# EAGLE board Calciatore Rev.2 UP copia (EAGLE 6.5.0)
Robot Calciatore SMD V2 Costruttori: Fabio Ricci Alessio Di Brigida
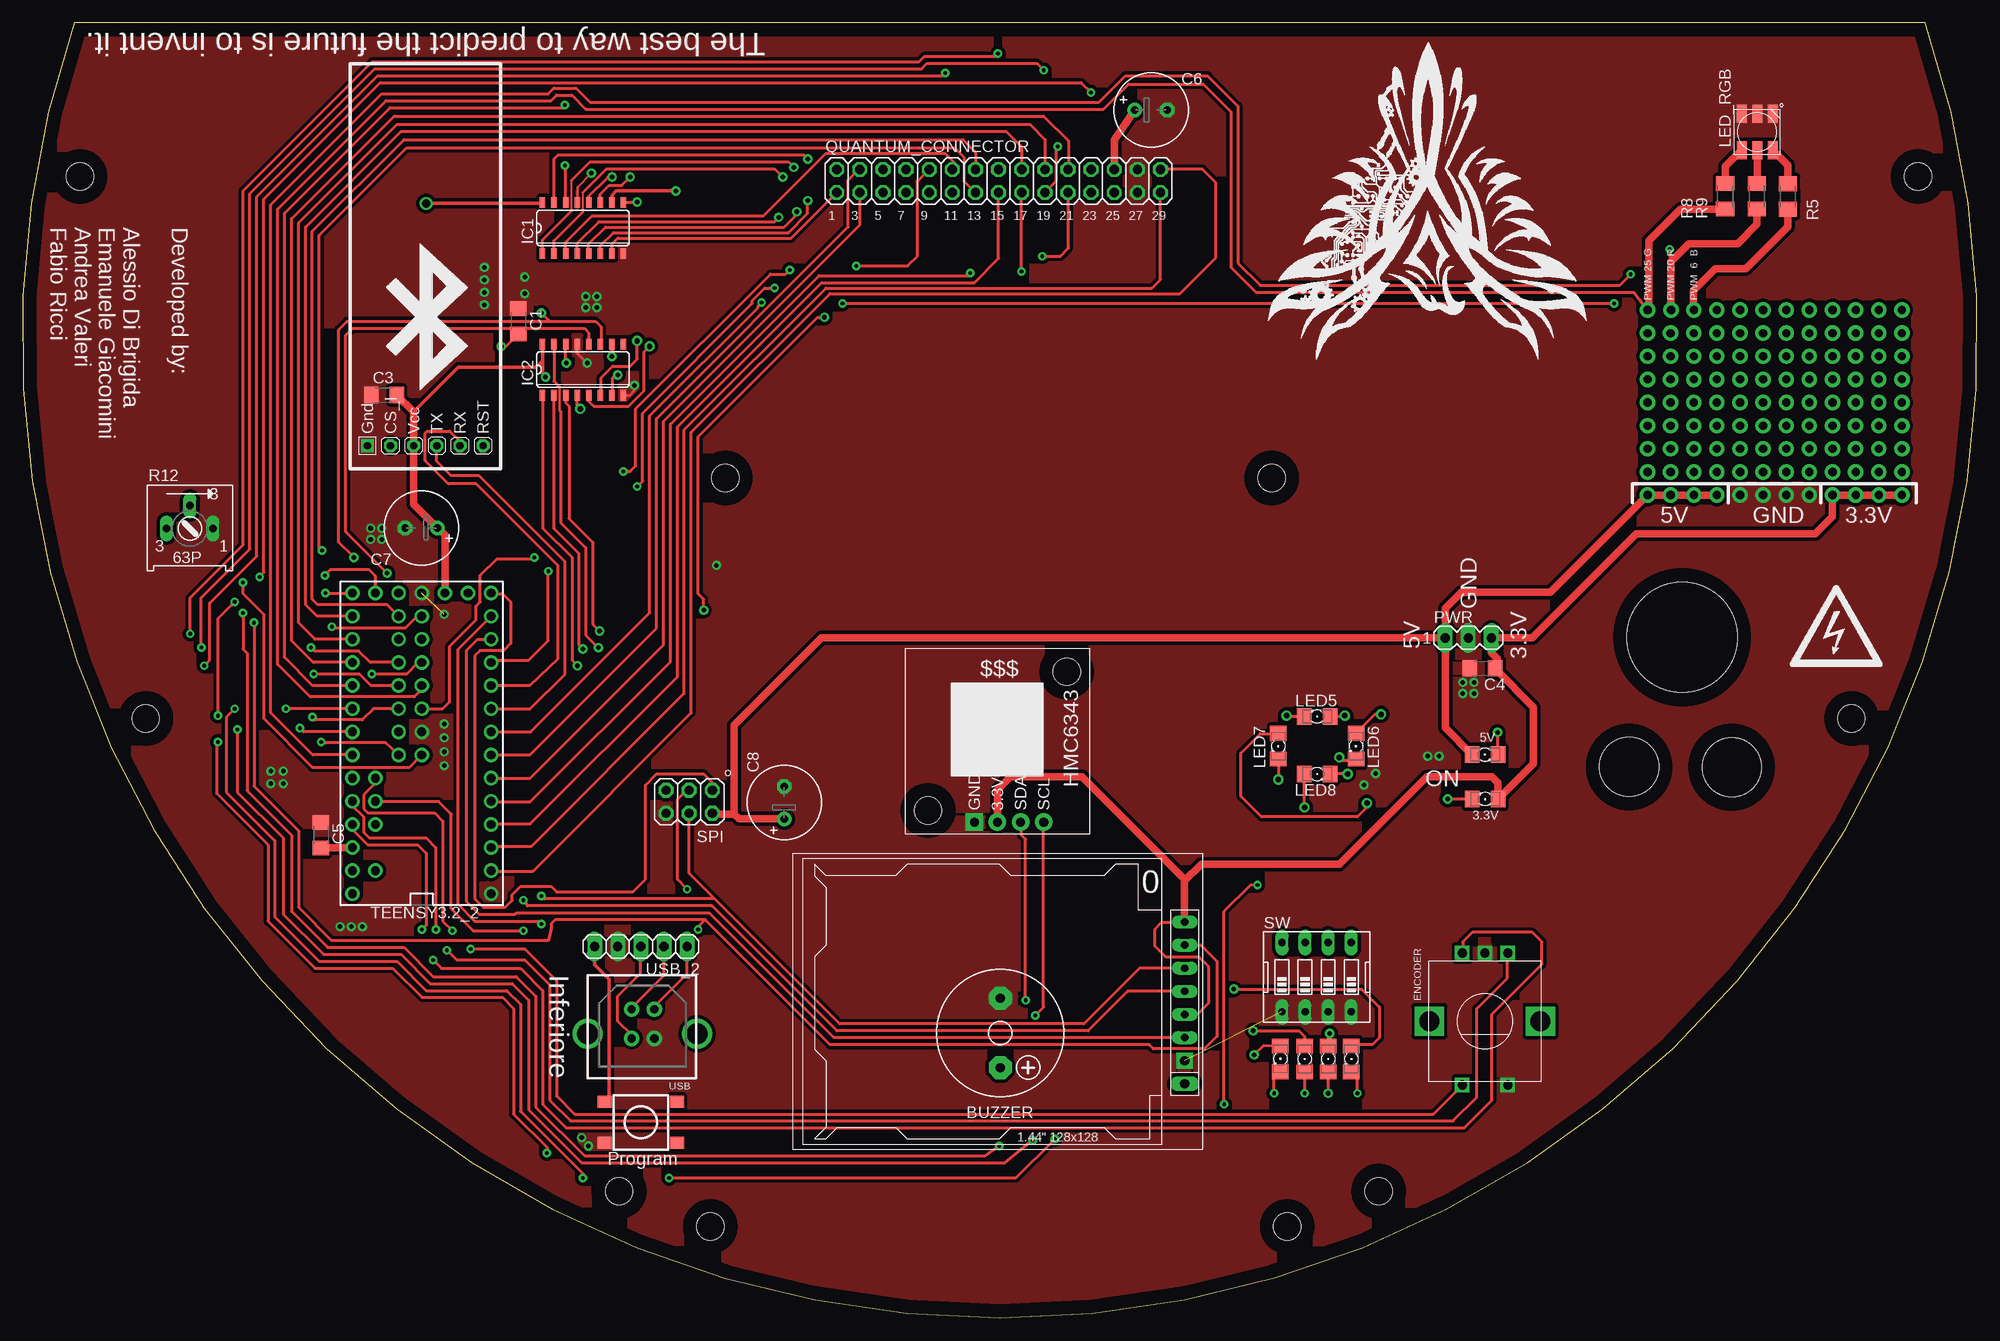
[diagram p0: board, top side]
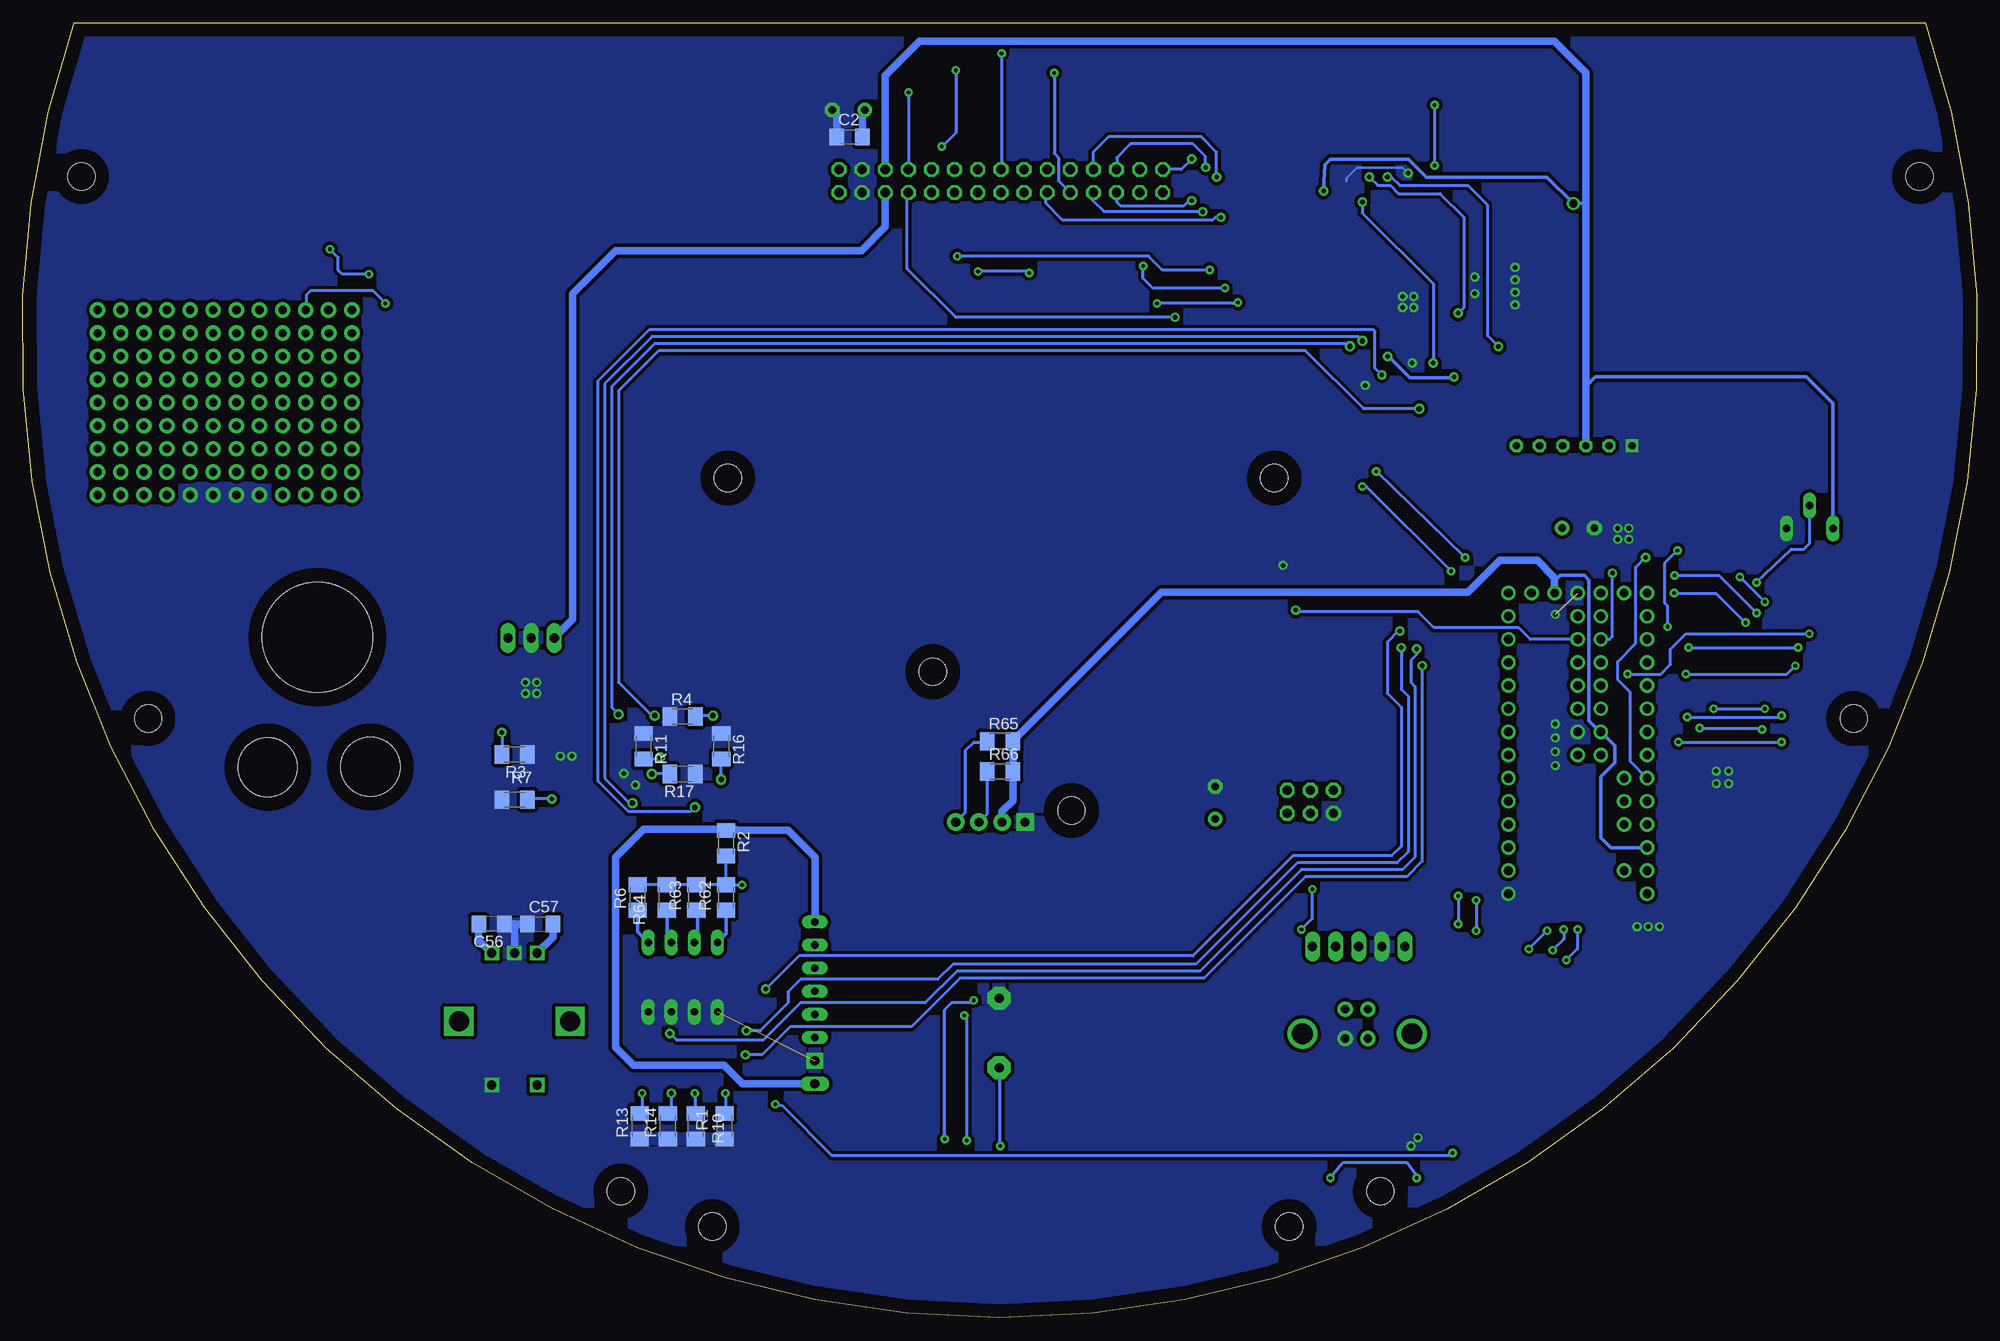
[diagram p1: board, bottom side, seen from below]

Size 214.58 x 142.18 mm. Coordinates in mm from the lower left corner, seen from the top.
Outline: 107.29,0.02 arc109 208.94,142.18 5.64,142.18 arc109 107.29,0
Copper layers (1*16): Top 0.035mm / dielectric 1.5mm / Bottom 0.035mm
Design rules "SparkFun *": minimum track width 6mil, minimum drill 8mil, track to track 6mil, track to pad 6mil, pad to pad 6mil, via to via 6mil, smd to smd 6mil, copper to edge 1.5mm, drill to drill 6mil, minimum pad ring 12mil, minimum via ring 10mil, stop-mask expansion 4mil, vias tented up to drill 25mil, thermal gap 0mil
Net classes: 0 default: width 0.254 mm, drill 0.254 mm, clearance 0.203 mm; 1 power: width 1.016 mm, drill 0.889 mm, clearance 0.508 mm; 2 gnd: width 0.864 mm, drill 0.406 mm, clearance 0.381 mm; 3 power usb: width 0.305 mm, drill 0.406 mm, clearance 0.203 mm
Holes 3 mm at 13.52,65.8 6.28,125.31 77.14,92.19 137.16,92.19 208.13,125.31 200.82,65.8 148.9,13.88 138.86,10.02 75.52,10.02 65.48,13.88
Holes 6.5 mm at 176.41,60.49 187.68,60.44
Holes 12.1 mm at 182.22,74.72

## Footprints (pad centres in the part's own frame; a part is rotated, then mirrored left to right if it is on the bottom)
F/CM12P = drill 1.016 pad 2.54 octagon: + 3.81,0; - -3.81,0
C1206 = smd 1.6 x 1.8: 1 -1.4,0; 2 1.4,0
E3,5-8 = drill 0.813 pad 1.6: + -1.778,0 | drill 0.813 pad 1.6 octagon: - 1.778,0
DISPLAY128X128 = drill 0.8 long: CS 20.32,-5.08; DC 20.32,0; LED 20.32,7.62; RST 20.32,-2.54; SCK 20.32,5.08; SDA 20.32,2.54 | drill 1 pad 1.778 square: GND 20.32,-7.62 | drill 1 long: VCC 20.32,-10.16
ALPS_EC12E_SW = drill 1 square: A -2.5,-7.5; B 2.5,-7.5; C 0,-7.5; D -2.5,7; E 2.5,7 | drill 2.2 square: GND1 -6.1,0; GND2 6.1,0
SO16 = smd 0.6 x 1.2: 1 -4.445,-2.8; 2 -3.175,-2.8; 3 -1.905,-2.8; 4 -0.635,-2.8; 5 0.635,-2.8; 6 1.905,-2.8; 7 3.175,-2.8; 8 4.445,-2.8; 9 4.445,2.8; 10 3.175,2.8; 11 1.905,2.8; 12 0.635,2.8; 13 -0.635,2.8; 14 -1.905,2.8; 15 -3.175,2.8; 16 -4.445,2.8
1206 = smd 1.6 x 1.803: A -1.422,0; C 1.422,0
RGBLED5050 = smd 2 x 1.1: 1 -2,1.7; 2 -2,0; 3 -2,-1.7; 4 2,-1.7; 5 2,0; 6 2,1.7
TACTILE_SWITCH_TALL = smd 1.55 x 1.3: A1 -3.975,-2.25; A2 3.975,-2.25; B1 -3.975,2.25; B2 3.975,2.25
MA03-1 = drill 1.016 long: 1 -2.54,0; 2 0,0; 3 2.54,0
2X15 = drill 1.016 octagon: 1 -17.78,-1.27; 2 -17.78,1.27; 3 -15.24,-1.27; 4 -15.24,1.27; 5 -12.7,-1.27; 6 -12.7,1.27; 7 -10.16,-1.27; 8 -10.16,1.27; 9 -7.62,-1.27; 10 -7.62,1.27; 11 -5.08,-1.27; 12 -5.08,1.27; 13 -2.54,-1.27; 14 -2.54,1.27; 15 0,-1.27; 16 0,1.27; 17 2.54,-1.27; 18 2.54,1.27; 19 5.08,-1.27; 20 5.08,1.27; 21 7.62,-1.27; 22 7.62,1.27; 23 10.16,-1.27; 24 10.16,1.27; 25 12.7,-1.27; 26 12.7,1.27; 27 15.24,-1.27; 28 15.24,1.27; 29 17.78,-1.27; 30 17.78,1.27
M1206 = smd 1.6 x 2: 1 -1.4,0; 2 1.4,0
S63P = drill 0.813 long: A 2.54,0; E -2.54,0; S 0,2.54
2X03 = drill 1.016 octagon: 1 -2.54,-1.27; 2 -2.54,1.27; 3 0,-1.27; 4 0,1.27; 5 2.54,-1.27; 6 2.54,1.27
EDG-04 = drill 0.813 long: 1 -3.81,-3.81; 2 -1.27,-3.81; 3 1.27,-3.81; 4 3.81,-3.81; 5 3.81,3.81; 6 1.27,3.81; 7 -1.27,3.81; 8 -3.81,3.81
TEENSY3_ALL_PINS_&_PADS = drill 0.965: 0 -7.62,13.97; 1 -7.62,11.43; 2 -7.62,8.89; 3 -7.62,6.35; 3.3V 7.62,11.43; 3.3V1 -2.54,-16.51; 3.3V2 2.54,-1.27; 4 -7.62,3.81; 5 -7.62,1.27; 6 -7.62,-1.27; 7 -7.62,-3.81; 8 -7.62,-6.35; 9 -7.62,-8.89; 10 -7.62,-11.43; 11 -7.62,-13.97; 12 -7.62,-16.51; 13 7.62,-16.51; 14/A0 7.62,-13.97; 15/A1 7.62,-11.43; 16/A2 7.62,-8.89; 17/A3 7.62,-6.35; 18/A4 7.62,-3.81; 19/A5 7.62,-1.27; 20/A6 7.62,1.27; 21/A7 7.62,3.81; 22/A8 7.62,6.35; 23/A9 7.62,8.89; 24 0,-3.81; 25 0,-6.35; 26 0,-8.89; 27 0,-11.43; 28 0,-13.97; 29 2.54,-13.97; 30 2.54,-11.43; 31 2.54,-8.89; 32 2.54,-6.35; 33 2.54,-3.81; A10 5.08,6.35; A11 5.08,3.81; A12 0,1.27; A13 2.54,1.27; AGND 7.62,13.97; AREF 5.08,8.89; GND -7.62,16.51; GND1 0,-16.51; GND2 0,-1.27; PGM 2.54,-16.51; RESET/DAC 5.08,-16.51; VBAT -5.08,-16.51; VIN 7.62,16.51; VUSB 5.08,13.97
HMC6343 = drill 1 pad 1.93: 3.3 10.16,1.27; SCL 15.24,1.27; SDA 12.7,1.27 | drill 1 pad 1.93 square: GND 7.62,1.27 | hole 3: 2.54,2.54; 17.78,17.78
BLUETOOTH = drill 0.8 pad 1.422 octagon: CS_I -3.81,-5.08; RST 6.35,-5.08; RX 3.81,-5.08; TX 1.27,-5.08; VCC -1.27,-5.08 | drill 0.8 pad 1.422 square: GND -6.35,-5.08
USB-B-PTH-VERTICAL = drill 0.914 pad 1.676: D+ 4.826,4.394; D- 4.826,7.595; GND 7.315,4.394; VBUS 7.315,7.595 | drill 2.286: P$1 0,4.902; P$2 12.04,4.902
1X05 = drill 1.016 long: 1 -5.08,0; 2 -2.54,0; 3 0,0; 4 2.54,0; 5 5.08,0

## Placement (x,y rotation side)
BUZZER  F/CM12P  [F/CM12P]  107.36,31.27 270 top
C1  [C1206]  54.44,109.41 270 top
C2  [C1206]  123.78,129.66 0 bottom
C3  [C1206]  39.68,101.31 0 top
C4  [C1206]  160.3,71.31 0 top
C5  [C1206]  32.74,53 270 top
C6  [E3,5-8]  123.9,132.6 0 top
C7  [E3,5-8]  43.77,86.71 180 top
C8  [E3,5-8]  83.62,56.56 90 top
C56  [C1206]  163.1,43.22 180 bottom
C57  [C1206]  157.76,43.22 0 bottom
DISPLAY1  DISPLAY128X128  [DISPLAY128X128]  107.28,35.84 0 top
ENCODER  EC12E_SW  [ALPS_EC12E_SW]  160.58,32.55 180 top
HIGHVOLTAGE  LOGO  [LOGOHV]  198.68,75 0 top
IC1  74LS595D  [SO16]  61.52,119.65 0 top
IC2  74LS595D  [SO16]  61.52,104.11 0 top
LED1  [1206]  140.77,28.41 270 top
LED2  [1206]  138.11,28.43 270 top
LED3  [1206]  143.36,28.41 270 top
LED4  [1206]  145.9,28.41 270 top
LED5  [1206]  142.14,66.01 180 top
LED6  [1206]  146.41,62.75 270 top
LED7  [1206]  137.87,62.75 270 top
LED8  [1206]  142.14,59.71 0 top
LED_3.3  [1206]  160.59,56.94 180 top
LED_5  [1206]  160.58,61.84 0 top
LED_RGB  [RGBLED5050]  190.47,130.19 90 top
PROGRAM  SWITCH-MOMENTARY-2SMD-4  [TACTILE_SWITCH_TALL]  67.87,21.45 180 top
PWR  [MA03-1]  158.75,74.64 0 top
QUANTUM_CONNECTOR  [2X15]  107.17,124.81 0 top
R1  1K  [M1206]  137.51,21.02 90 bottom
R2  10K  [M1206]  137.34,52.11 270 bottom
R3  1K  [M1206]  160.58,61.84 180 bottom
R4  1K  [M1206]  142.14,66.01 0 bottom
R5  1K  [M1206]  193.83,123.11 270 top
R6  10K  [M1206]  147.07,46.14 90 bottom
R7  1K  [M1206]  160.56,56.89 0 bottom
R8  1K  [M1206]  186.95,123.11 270 top
R9  1K  [M1206]  190.44,123.13 270 top
R10  1K  [M1206]  140.67,21.02 90 bottom
R11  1K  [M1206]  146.41,62.75 270 bottom
R12  [S63P]  18.34,86.66 0 top
R13  1K  [M1206]  146.84,21.02 90 bottom
R14  1K  [M1206]  143.74,21.02 90 bottom
R16  1K  [M1206]  137.87,62.75 270 bottom
R17  1K  [M1206]  142.14,59.71 180 bottom
R62  10K  [M1206]  137.34,46.14 90 bottom
R63  10K  [M1206]  140.62,46.14 270 bottom
R64  10K  [M1206]  143.84,46.14 270 bottom
R65  3.3K  [M1206]  107.27,63.31 0 bottom
R66  3.3K  [M1206]  107.24,59.99 0 bottom
SPI  [2X03]  73.18,56.66 180 top
SW  [EDG-04]  142.09,37.41 0 top
TEENSY3.2_2  TEENSY_3.1_ALL_PINS_AND_PADS  [TEENSY3_ALL_PINS_&_PADS]  43.82,63.06 180 top
U$1  [PHOENIX]  153.96,119.77 180 top
U$5  HMC6343  [HMC6343]  96.88,53.15 0 top
U$9  BLUETOOTH  [BLUETOOTH]  44.2,100.83 0 top
USB  USBPTH-VERTICAL  [USB-B-PTH-VERTICAL]  62.03,26.28 0 top
USB_2  [1X05]  67.87,40.76 180 top

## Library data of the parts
BUZZER = buzzer; OC_FARNELL: unknown; OC_NEWARK: unknown
C1-C5 C56 C57 R2 R6 R62-R66 = rcl
C6-C8 LED1-LED8 LED_3.3 LED_5 LED_RGB = adafruit
DISPLAY1 = Display 128x128
ENCODER = switch-alps; MPN: EC12E2424407; OC_FARNELL: 1520813; OC_NEWARK: 74M1068
HIGHVOLTAGE = Loghi
IC1 IC2 = SparkFun-DigitalIC; PROD_ID: IC-07875
PROGRAM = SparkFun-Electromechanical; PROD_ID: SWCH-11966
PWR = con-lstb; OC_FARNELL: unknown; OC_NEWARK: unknown
QUANTUM_CONNECTOR SPI USB_2 = pinhead
R1 R3-R5 R7-R11 R13 R14 R16 R17 = resistor
R12 = pot
SW = special
TEENSY3.2_2 = Teensy_3_and_LC_Series_Boards_v1.1
U$1 = Phoenix
U$5 = HMC6343
U$9 = Bluetooth
USB = SparkFun-Connectors

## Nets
3.3V [power]: C2.2 C3.2 C4.2 C5.2 C6.+ C7.+ DISPLAY1.LED DISPLAY1.RST DISPLAY1.VCC IC1.10 IC1.16 IC2.10 IC2.16 LED_3.3.A PWR.3 QUANTUM_CONNECTOR.26 R2.1 R12.E R65.2 R66.2 TEENSY3.2_2.3.3V TEENSY3.2_2.3.3V1 TEENSY3.2_2.3.3V2 U$5.3.3 U$9.VCC
5V [power]: C8.+ LED_5.A PWR.1 QUANTUM_CONNECTOR.25 SPI.2
AGND: TEENSY3.2_2.AGND
AREF: TEENSY3.2_2.AREF
BLUE: R5.2 TEENSY3.2_2.6
BT-RX_TEENSY-TX: TEENSY3.2_2.8 U$9.RX
BT-TX_TEENSY-RX: TEENSY3.2_2.7 U$9.TX
CLOCK: IC1.11 IC2.11 TEENSY3.2_2.21/A7
CS: DISPLAY1.CS TEENSY3.2_2.10
D+: USB.D+ USB_2.3
D-: USB.D- USB_2.2
DATA-IN: IC1.14 TEENSY3.2_2.17/A3
DATA-OUT: IC1.9 IC2.14
DC: DISPLAY1.DC TEENSY3.2_2.A10
DIPSW: R2.2 R6.2 R62.2 R63.1 R64.1 TEENSY3.2_2.A13
DIR: C56.2 ENCODER.A TEENSY3.2_2.22/A8
GND [gnd]: BUZZER.- C1.1 C2.1 C3.1 C4.1 C5.1 C6.- C7.- C8.- C56.1 C57.1 DISPLAY1.GND ENCODER.C ENCODER.D IC1.8 IC1.13 IC2.8 IC2.13 LED_RGB.4 LED_RGB.5 LED_RGB.6 PROGRAM.B2 PWR.2 QUANTUM_CONNECTOR.27 QUANTUM_CONNECTOR.28 R1.1 R3.1 R4.1 R7.1 R10.1 R11.1 R12.A R13.1 R14.1 R16.1 R17.1 SPI.6 SW.1 SW.2 SW.3 SW.4 TEENSY3.2_2.GND TEENSY3.2_2.GND1 TEENSY3.2_2.GND2 U$5.GND U$9.GND USB.GND USB_2.4
GREEN: R8.2 TEENSY3.2_2.25
INA1: IC1.15 QUANTUM_CONNECTOR.2
INA2: IC1.2 QUANTUM_CONNECTOR.8
INA3: IC1.4 QUANTUM_CONNECTOR.11
INA4: IC1.6 QUANTUM_CONNECTOR.5
INB1: IC1.1 QUANTUM_CONNECTOR.6
INB2: IC1.3 QUANTUM_CONNECTOR.12
INB3: IC1.5 QUANTUM_CONNECTOR.7
INB4: IC1.7 QUANTUM_CONNECTOR.1
LATCH: C1.2 IC1.12 IC2.12 TEENSY3.2_2.30
LED1: IC2.15 LED1.A
LED2: IC2.1 LED2.A
LED3: IC2.2 LED3.A
LED4: IC2.3 LED4.A
LED5: IC2.4 LED5.A
LED6: IC2.5 LED6.A
LED7: IC2.6 LED7.A
LED8: IC2.7 LED8.A
LED_3.3: LED_3.3.C R7.2
LINEA1: QUANTUM_CONNECTOR.15 TEENSY3.2_2.2
LINEA2: QUANTUM_CONNECTOR.17 TEENSY3.2_2.3
LINEA3: QUANTUM_CONNECTOR.19 TEENSY3.2_2.31
LINEA4: QUANTUM_CONNECTOR.21 TEENSY3.2_2.24
LINEA5: QUANTUM_CONNECTOR.23 TEENSY3.2_2.27
LINEA6: QUANTUM_CONNECTOR.16 TEENSY3.2_2.26
LINEA7: QUANTUM_CONNECTOR.18 TEENSY3.2_2.14/A0
LINEA8: QUANTUM_CONNECTOR.20 TEENSY3.2_2.15/A1
LINEA9: QUANTUM_CONNECTOR.22 TEENSY3.2_2.16/A2
LINEAANT: QUANTUM_CONNECTOR.24 TEENSY3.2_2.33
MISO: SPI.1 TEENSY3.2_2.12
MOSI: DISPLAY1.SDA SPI.4 TEENSY3.2_2.11
N$1: LED2.C R1.2
N$2: LED_5.C R3.2
N$3: LED5.C R4.2
N$4: TEENSY3.2_2.VUSB
N$5: LED6.C R11.2
N$6: LED7.C R16.2
N$8: LED_RGB.3 R5.1
N$10: LED_RGB.1 R8.1
N$11: LED_RGB.2 R9.1
N$12: LED1.C R10.2
N$13: LED4.C R13.2
N$14: LED3.C R14.2
N$16: LED8.C R17.2
N$18: R64.2 SW.6
N$20: R62.1 SW.8
N$96: R6.1 SW.5
N$97: R63.2 SW.7
PALLA: QUANTUM_CONNECTOR.13 TEENSY3.2_2.28
PROGRAM: PROGRAM.A2 USB_2.5
PULS: C57.2 ENCODER.B TEENSY3.2_2.23/A9
PWM1: QUANTUM_CONNECTOR.4 TEENSY3.2_2.5
PWM2: QUANTUM_CONNECTOR.10 TEENSY3.2_2.9
PWM3: QUANTUM_CONNECTOR.9 TEENSY3.2_2.32
PWM4: QUANTUM_CONNECTOR.3 TEENSY3.2_2.4
RED: R9.2 TEENSY3.2_2.20/A6
RESET: SPI.5
SCK: DISPLAY1.SCK SPI.3 TEENSY3.2_2.13
SCL: R65.1 TEENSY3.2_2.19/A5 U$5.SCL
SDA: R66.1 TEENSY3.2_2.18/A4 U$5.SDA
SEL: ENCODER.E TEENSY3.2_2.A11
SOLENOIDE: QUANTUM_CONNECTOR.14 TEENSY3.2_2.29
SPEED: R12.S TEENSY3.2_2.A12
TEENSY1-RX_TEENSY2-TX: QUANTUM_CONNECTOR.29 TEENSY3.2_2.1
TEENSY1-TX_TEENSY2-RX: QUANTUM_CONNECTOR.30 TEENSY3.2_2.0
TONE: BUZZER.+ TEENSY3.2_2.RESET/DAC
VBATTEENSY: TEENSY3.2_2.VBAT
VIN: TEENSY3.2_2.VIN
VUSB: USB.VBUS USB_2.1

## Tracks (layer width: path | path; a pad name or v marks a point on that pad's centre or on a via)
3.3V  (via drill 0.51, 0.89, 0.9 pad 1.68)
  Top 0.305: DISPLAY1.RST 129,33.3 130.25,34.56 130.25,38.52 129.19,39.59 125.53,39.59 124.31,40.81 124.31,42.64 125.07,43.4 127.54,43.4 DISPLAY1.LED
  Top 0.406: 42.93,99.46 47.83,104.36 56.34,104.36 57.08,105.1 IC2.16 57.08,103.62 v57.41,103.29 | IC1.16 56.97,122.34 v44.3,122.34 | IC1.10 64.72,122.48 64.72,123.26 65.18,123.71 v71.73,123.71 | 64.72,106.88 IC2.10 v64.7,105.53
  Top 0.813: TEENSY3.2_2.3.3V1 46.36,85.89 C7.+ 42.93,89.32 U$9.VCC 42.93,99.46 C3.2 41.23,101.46 | TEENSY3.2_2.3.3V 32.77,51.63 C5.2 | QUANTUM_CONNECTOR.26 119.87,129.33 C6.+ | U$5.3.3 107.04,57.98 108.46,59.4 116.32,59.4 127.6,48.12 127.6,47.97 | 127.6,47.97 DISPLAY1.LED | 127.6,47.97 129.43,49.8 144.58,49.8 154.18,59.4 161.34,59.4 162.02,58.73 LED_3.3.A 165.92,60.84 165.92,67.02 161.7,71.23 C4.2 161.95,71.57 161.95,72.36 161.29,73.02 PWR.3 165.76,74.64 177.19,86.07 196.88,86.07 198.75,87.94 v198.75,90.33 v201.29,90.33 v203.83,90.33 v206.37,90.33
  Bottom 0.406: 42.93,122.34 v44.3,122.34 47.2,125.24 60.46,125.24 62.44,127.22 70.97,127.22 71.58,126.61 v71.73,123.71 | R12.E 15.8,100.4 18.7,103.29 41.86,103.29 42.93,102.23 | TEENSY3.2_2.3.3V 40.19,51.63 41.25,52.7 41.25,59.4 39.73,60.93 39.73,62.78 TEENSY3.2_2.3.3V2 41.38,64.33 42.57,65.52 42.57,80.99 43.08,81.5 45.75,81.5 46.36,80.89 TEENSY3.2_2.3.3V1 | v57.41,103.29 57.48,103.22 62.26,103.22 64.57,105.53 v64.7,105.53
  Bottom 0.813: C2.2 122.38,132.35 C6.+ | QUANTUM_CONNECTOR.26 119.87,136.39 116.11,140.15 46.41,140.15 42.93,136.67 42.93,122.34 42.93,102.23 U$9.VCC | R2.1 136.2,53.51 | 136.2,53.51 130.55,53.51 127.6,50.56 DISPLAY1.LED | DISPLAY1.VCC 135.55,25.68 137.57,27.7 147.48,27.7 149.46,29.68 149.46,50.56 146.41,53.61 136.3,53.61 136.2,53.51 | TEENSY3.2_2.3.3V1 46.36,81.27 48.26,83.18 52.38,83.18 55.88,79.67 89.51,79.67 R65.2 105.84,63.29 R66.2 105.84,56.79 107.04,55.59 U$5.3.3
5V  (via drill 0.9 pad 1.68)
  Top 0.813: PWR.1 156.21,77.89 157.99,79.67 167.77,79.67 v178.43,90.33 v180.97,90.33 v183.51,90.33 v186.05,90.33 | PWR.1 87.73,74.64 78.13,65.04 78.13,55.29 | 78.13,55.29 75.82,55.29 SPI.2 | C8.+ 78.64,54.78 78.13,55.29 | PWR.1 156.21,64.79 LED_5.A
  Bottom 0.813: QUANTUM_CONNECTOR.25 119.87,119.78 122.48,117.16 149.46,117.16 154.18,112.44 154.18,76.67 PWR.1
BLUE  (via drill 0.41 pad 0.81, 0.9 pad 1.68)
  Top 0.305: v81.13,111.47 80.72,111.07 80.72,110.91 68.84,99.03 68.84,77.38 55.78,64.33 TEENSY3.2_2.6 | v90.02,111.37 v174.76,111.37
  Top 0.813: R5.2 193.83,119.77 189.23,115.18 185.88,115.18 183.44,112.74 183.44,110.71 v183.51,110.65
  Bottom 0.305: v81.13,111.47 81.49,111.52 81.64,111.37 v90.02,111.37 | v174.76,111.37 176.13,112.74 182.98,112.74 183.44,112.28 183.44,110.71 v183.51,110.65
BT-RX_TEENSY-TX
  Top 0.305: TEENSY3.2_2.8 51.49,69.46 55.73,69.46 58.78,72.36 58.78,82.57 49.79,91.56 46.74,91.56 44.2,94.1 44.2,97.1 44.45,97.35 46.89,97.35 48.01,96.23 U$9.RX
BT-TX_TEENSY-RX
  Top 0.305: TEENSY3.2_2.7 55.73,66.87 59.54,70.68 59.54,83.02 50.09,92.47 47.04,92.47 45.47,94.05 U$9.TX
CLOCK  (via drill 0.51)
  Top 0.305: v36.38,83.48 34.7,85.16 34.7,108.47 35.61,109.39 57.89,109.39 | 57.89,109.39 62.89,109.39 63.5,108.78 63.5,106.98 IC2.11 | IC1.11 63.43,123.33 64.42,124.32 65.79,124.32 v66.7,125.24 | v56.95,110.3 57.89,109.39
  Bottom 0.305: TEENSY3.2_2.21/A7 36.22,59.25 38.05,61.08 38.05,68.7 39.42,70.07 39.42,72.05 37.44,74.03 37.44,82.41 v36.38,83.48 | v66.7,125.24 65.79,124.32 64.42,124.32 63.5,123.41 58.93,123.41 56.34,120.82 56.34,110.91 v56.95,110.3
CS
  Top 0.305: DISPLAY1.CS 89.09,30.76 75.39,44.47 54.21,44.47 54.05,44.31 50.09,44.31 48.72,45.69 48.72,73.27 49.94,74.49 TEENSY3.2_2.10
D+
  Top 0.305: USB.D+ 66.86,31.06 65.33,32.58 65.33,35.32 67.85,37.84 67.85,40.73 USB_2.3
D-
  Top 0.305: USB.D- 66.86,34.03 70.41,37.58 USB_2.2
DATA-IN  (via drill 0.41 pad 0.81)
  Top 0.305: TEENSY3.2_2.17/A3 31.85,69.41 28.76,72.51 28.76,121.28 40.34,132.86 59.54,132.86 v59.54,133.16 | v59.54,126.51 59.54,122.53 IC1.14
  Bottom 0.305: v59.54,133.16 v59.54,126.51
DATA-OUT  (via drill 0.51)
  Top 0.305: IC1.9 67.42,122.45 v67.47,122.5 | v59.69,104.82 59.62,104.89 IC2.14
  Bottom 0.305: v67.47,122.5 67.47,121.28 59.69,113.5 v59.69,104.82
DC  (via drill 0.41 pad 0.81)
  Top 0.305: DISPLAY1.DC 121.33,35.84 117,31.51 89.41,31.51 75.7,45.23 55.43,45.23 v54.97,45.84 | TEENSY3.2_2.A10 38.79,56.66 45.67,56.66 47.04,55.29 47.04,44.92 49.48,42.49 v54.97,42.49
  Bottom 0.305: v54.97,45.84 v54.97,42.49
DIPSW  (via drill 0.41)
  Top 0.305: TEENSY3.2_2.A13 39.86,63.11 33.28,63.11 v32.77,63.21 | v21.44,63.21 21.29,63.06 21.29,57.57 26.93,51.93 26.93,43.55 32.11,38.37 40.64,38.37 43.84,35.17 52.68,35.17 53.9,33.95 53.9,22.37 57.56,18.71 v57.56,18.1 | v131.93,23.44 131.93,44.62 134.83,47.51 v135.59,47.51
  Bottom 0.305: v32.77,63.21 v21.44,63.21 | v57.56,18.1 57.86,17.8 125.68,17.8 131.17,23.28 v131.93,23.44 | v135.59,47.51 137.31,47.51 R62.2 | R62.2 R63.1 R64.1 | R64.1 144.3,47.54 144.43,47.67 143.97,47.67 R64.1 | R64.1 R6.2 | R62.2 R2.2
DIR  (via drill 0.41)
  Top 0.305: TEENSY3.2_2.22/A8 36.2,56.23 37.44,54.98 37.44,53.31 38.05,52.7 44.3,52.7 45.37,51.63 v45.37,42.64 | v46.59,40.35 47.65,39.28 55.12,39.28 57.86,36.54 57.86,23.89 60.15,21.61 157.08,21.61 159.67,24.2 159.67,33.95 163.02,37.3 163.02,39.99 ENCODER.A
  Bottom 0.305: v45.37,42.64 45.37,41.57 v46.59,40.35
  Bottom 0.813: ENCODER.A 164.5,41.47 C56.2
GND  (via drill 0.5, 0.51, 0.9 pad 1.68)  (2 unrouted)
  Top 0.254: IC1.13 60.91,122.48 60.91,124.15 v62.44,125.67
  Top 0.305: IC2.8 66.7,101.31 67.16,101.77 v67.16,102.38 | v61.98,104.82 60.89,105.91 IC2.13
  Bottom 0.254: v62.44,125.67 63.05,126.28 68.08,126.28 69.24,125.11 69.24,124.81
  Bottom 0.813: ENCODER.C 160.58,43.25 161.67,43.25 C56.1 C57.1 | C2.1 125.18,132.1 C6.-
  other vias: 188.59,90.33 191.13,90.33 193.67,90.33 196.21,90.33 27.23,60.01 28.6,60.01 46.28,65.19 46.28,63.67 46.28,62.14 46.28,60.62 27.23,58.64 28.6,58.64 46.28,77.23 50.7,111.22 50.7,112.59 55.12,114.27 55.12,112.44 50.7,113.96 50.7,115.33 61.83,110.91 61.83,112.13 63.05,112.13 63.05,110.91 158.14,68.55 159.36,68.55 159.36,69.76 158.14,69.76 61.37,19.78 62.13,18.86 34.85,42.94 36.07,42.94 37.29,42.94 39.42,86.68 38.2,86.68 38.2,85.46 39.42,85.46 148.57,59.76 155.55,61.66 154.28,61.66 147.3,58.49 76.18,82.62
  pour Bottom: -15.21,153.38 230.53,153.38 230.53,-13.62 -15.85,-13.62 -15.85,153.38
  pour Top: -15.85,153.38 230.53,153.38 230.53,-0.29 230.53,-13.62 -15.85,-13.62
GREEN  (via drill 0.9 pad 1.68)
  Top 0.305: TEENSY3.2_2.25 43.82,68.98 43.01,68.16 31.58,68.16 27.99,71.75 27.99,121.73 39.88,133.62 58.02,133.62 58.63,134.23 60.3,134.23 61.83,132.71 118.67,132.71 121.42,135.45 129.64,135.45 132.69,132.4 132.69,115.33 135.44,112.59 176.94,112.59 v178.43,110.65
  Top 0.813: R8.2 182.05,121.71 178.57,118.23 178.57,110.79 v178.43,110.65
INA1  (via drill 0.51)
  Top 0.305: IC1.15 58.35,127.24 58.78,127.68 85.75,127.68 v86.21,127.22
  Bottom 0.305: v86.21,127.22 87.35,126.08 QUANTUM_CONNECTOR.2
INA2  (via drill 0.51)
  Top 0.229: 61.52,121.43 61.52,123.56
  Top 0.305: IC1.2 58.35,118.25 61.52,121.43 | v83.47,125.24 82.55,126.15 64.11,126.15 61.52,123.56
  Bottom 0.305: v83.47,125.24 83.47,127.98 85.14,129.66 95.35,129.66 97.03,127.98 97.03,126.1 QUANTUM_CONNECTOR.8
INA3  (via drill 0.51)
  Top 0.305: IC1.4 60.89,117.97 63.27,120.36 82.55,120.36 v83.01,120.82
  Bottom 0.305: v83.01,120.82 83.62,120.82 83.92,120.51 100.38,120.51 102.21,122.34 102.21,123.41 QUANTUM_CONNECTOR.11
INA4  (via drill 0.51)
  Top 0.305: IC1.6 63.43,117.69 64.87,119.14 84.08,119.14 86.21,121.28 v86.21,122.65
  Bottom 0.305: v86.21,122.65 86.52,122.65 87.13,122.04 93.98,122.04 94.44,122.5 94.44,123.51 QUANTUM_CONNECTOR.5
INB1  (via drill 0.51)
  Top 0.229: 60.25,121.53 60.25,124.88
  Top 0.305: IC1.1 57.08,118.35 60.25,121.53 | 60.25,124.88 62.28,126.91 84.08,126.91 v84.69,126.31
  Bottom 0.305: v84.69,126.31 84.69,127.52 86.06,128.9 92.92,128.9 94.44,127.37 94.44,126.1 QUANTUM_CONNECTOR.6
INB2
  Top 0.305: IC1.3 59.62,118.08 62.51,120.97 81.33,120.97 88.19,127.83 101.3,127.83 102.21,126.91 102.21,126.2 QUANTUM_CONNECTOR.12
INB3  (via drill 0.51)
  Top 0.305: IC1.5 62.16,117.92 63.99,119.75 83.62,119.75 85.14,121.28 v84.99,121.43
  Bottom 0.305: v84.99,121.43 95.81,121.43 97.03,122.65 97.03,123.51 QUANTUM_CONNECTOR.7
INB4
  Top 0.305: IC1.7 64.7,117.9 65.33,118.53 84.38,118.53 QUANTUM_CONNECTOR.1
LATCH  (via drill 0.51)
  Top 0.305: v40.01,81.75 35.46,86.3 35.46,107.86 36.22,108.63 54.51,108.63 | 54.51,108.63 61.67,108.63 62.13,108.17 62.13,106.93 IC2.12 | 54.51,108.63 54.44,108.55 C1.2 53.07,106.65 v52.53,106.65 | IC1.12 62.16,123.13 64.27,125.24 v64.72,125.24
  Bottom 0.305: TEENSY3.2_2.30 40.34,74.49 40.01,74.82 v40.01,81.75 | v64.72,125.24 64.27,125.24 63.35,124.32 55.88,124.32 53.75,122.19 53.75,107.86 v52.53,106.65
LED1  (via drill 0.51)
  Top 0.254: 58.98,102.18 58.98,99.58
  Top 0.305: IC2.15 58.35,102.81 58.98,102.18 | 58.98,99.58 59.08,99.48 59.08,87.29 61.83,84.55 61.83,74.95 v63.2,73.57 | v135.13,31.51 140.16,31.51 140.77,30.9 LED1.A
  Bottom 0.305: v63.2,73.57 63.2,69 62.44,68.24 62.44,51.17 63.66,49.95 74.63,49.95 85.75,38.83 112.42,38.83 114.1,37.15 129.19,37.15 130.56,35.78 130.56,34.56 133.61,31.51 v135.13,31.51
LED2  (via drill 0.51)
  Top 0.305: IC2.1 57.1,101.28 57.1,86.68 60.3,83.48 60.3,72.2 v60.91,71.59 | v135.23,28.87 136.28,29.91 LED2.A
  Bottom 0.305: v60.91,71.59 60.91,50.11 62.59,48.43 73.71,48.43 84.84,37.3 111.66,37.3 117,31.97 130.31,31.97 133.4,28.87 v135.23,28.87
LED3  (via drill 0.51)
  Top 0.305: v61.52,73.42 61.06,73.88 61.06,83.94 58.35,86.66 IC2.2 | LED3.A 143.36,31.06 v143.51,31.21
  Bottom 0.305: v61.52,73.42 61.52,72.81 62.13,72.2 62.13,69.76 61.67,69.31 61.67,50.56 63.05,49.19 74.17,49.19 85.3,38.07 111.97,38.07 115.47,34.56 129.19,34.56 133.3,30.45 142.75,30.45 v143.51,31.21
LED4  (via drill 0.51)
  Top 0.305: IC2.3 59.62,100.47 60,100.09 60,87.75 62.59,85.16 62.59,76.17 v63.35,75.4 | v133,36.08 147.02,36.08 149,34.1 149,30.75 148.24,29.99 146.05,29.99 LED4.A
  Bottom 0.305: v63.35,75.4 63.5,75.4 64.72,74.18 64.72,68.55 63.2,67.02 63.2,51.78 64.27,50.71 75.09,50.71 86.06,39.74 129.34,39.74 v133,36.08
LED5  (via drill 0.6)
  Top 0.305: v145.19,66.11 145.09,66.01 LED5.A | 60.99,101.2 IC2.4 60.89,100.12 v61.22,99.79
  Bottom 0.305: v61.22,99.79 67.31,99.79 73.71,106.19 144.73,106.19 149.15,101.77 149.15,69.76 145.49,66.11 v145.19,66.11
LED6  (via drill 0.6)
  Top 0.305: v68.84,106.65 68.23,106.04 68.23,101.77 66.55,100.09 62.69,100.09 62.16,100.63 IC2.5 | v149.15,66.26 148.49,66.26 LED6.A
  Bottom 0.305: v68.84,106.65 69.14,106.95 145.19,106.95 149.91,102.23 149.91,67.02 v149.15,66.26
LED7  (via drill 0.6)
  Top 0.305: v147.63,56.51 147.63,56.05 146.56,54.98 136.05,54.98 133.76,57.27 133.76,61.99 135.89,64.13 137.82,64.13 LED7.A | IC2.6 63.53,101.41 63.53,103.22 64.8,104.49 66.7,104.49 67.47,105.25 v67.47,107.26
  Bottom 0.305: v67.47,107.26 67.92,107.71 145.49,107.71 150.68,102.53 150.68,59.25 147.78,56.35 v147.63,56.51
LED8  (via drill 0.51, 0.6)
  Top 0.305: v140.77,56.05 140.77,59.66 LED8.A | IC2.7 64.8,101.41 64.8,103.22 65.1,103.52 v65.33,103.52
  Bottom 0.305: v140.77,56.05 141.23,55.59 148.09,55.59 151.44,58.94 151.44,102.84 145.8,108.47 66.25,108.47 66.07,108.3 66.07,104.26 v65.33,103.52
LED_3.3  (via drill 0.51)
  Top 0.305: LED_3.3.C 156.49,56.94 v156.47,56.96
  Bottom 0.305: v156.47,56.96 159.08,56.96 R7.2
LINEA1
  Top 0.305: TEENSY3.2_2.2 51.49,54.22 55.73,54.22 71.89,70.37 71.89,97.81 87.73,113.66 104.5,113.66 107.17,116.32 QUANTUM_CONNECTOR.15
LINEA2  (via drill 0.41 pad 0.81)
  Top 0.305: TEENSY3.2_2.3 51.49,56.66 55.73,56.66 71.12,72.05 71.12,98.11 87.43,114.42 103.89,114.42 104.04,114.57 v104.04,114.72 | v109.68,114.88 109.71,114.9 QUANTUM_CONNECTOR.17
  Bottom 0.305: v104.04,114.72 104.19,114.88 v109.68,114.88
LINEA3  (via drill 0.41)
  Top 0.305: TEENSY3.2_2.31 38.15,71.95 36.91,73.19 32.03,73.19 v31.65,73.57 | v19.61,73.57 19.61,79.06 24.95,84.4 24.95,123.41 38.66,137.13 98.71,137.13 99.32,137.74 111.36,137.74 v112.12,136.97 | v113.64,128.59 113.49,128.44 113.49,124.78 QUANTUM_CONNECTOR.19
  Bottom 0.305: v31.65,73.57 v19.61,73.57 | v112.12,136.97 112.12,130.12 v113.64,128.59
LINEA4  (via drill 0.41)
  Top 0.305: TEENSY3.2_2.24 46.13,66.87 46.89,67.63 46.89,73.73 49.79,76.62 49.79,78.15 50.24,78.6 50.24,81.5 52.07,83.33 56.04,83.33 v56.19,83.48 | v65.94,92.93 66.7,92.93 67.31,93.54 67.31,99.79 82.1,114.57 83.77,114.57 v84.23,115.03 | v111.97,116.55 113.95,116.55 114.86,117.47 114.86,123.46 QUANTUM_CONNECTOR.21
  Bottom 0.305: v56.19,83.48 v65.94,92.93 | v84.23,115.03 89.41,115.03 90.94,116.55 v111.97,116.55
LINEA5  (via drill 0.51)
  Top 0.305: v74.78,77.69 74.78,78.91 74.17,79.52 74.17,96.74 87.28,109.85 v88.04,109.85
  Bottom 0.305: TEENSY3.2_2.27 49.03,74.49 50.3,75.76 59.59,75.76 61.37,77.54 74.63,77.54 v74.78,77.69 | QUANTUM_CONNECTOR.23 117.45,123.41 117.45,115.18 112.12,109.85 v88.04,109.85
LINEA6  (via drill 0.41)
  Top 0.305: TEENSY3.2_2.26 43.44,71.95 42.17,70.68 v38.36,70.68 | v18.39,75.1 18.39,79.06 24.18,84.85 24.18,123.71 38.36,137.89 98.4,137.89 99.01,138.5 106.78,138.5 v107.09,138.8
  Bottom 0.305: v38.36,70.68 34.7,70.68 33.63,71.75 33.63,73.42 31.96,75.1 v18.39,75.1 | v107.09,138.8 107.09,126.15 QUANTUM_CONNECTOR.16
LINEA7
  Top 0.305: TEENSY3.2_2.14/A0 32.31,77.03 31.04,78.3 31.04,119.75 41.56,130.27 108,130.27 109.68,128.59 109.68,126.1 QUANTUM_CONNECTOR.18
LINEA8
  Top 0.305: TEENSY3.2_2.15/A1 32.11,74.49 30.28,76.32 30.28,120.21 41.1,131.03 110.59,131.03 112.27,129.35 112.27,126.1 QUANTUM_CONNECTOR.20
LINEA9
  Top 0.305: TEENSY3.2_2.16/A2 31.91,71.95 29.52,74.34 29.52,120.67 40.8,131.94 112.12,131.94 114.86,129.2 114.86,126.15 QUANTUM_CONNECTOR.22
LINEAANT  (via drill 0.41)
  Top 0.305: TEENSY3.2_2.33 38.51,66.87 37.29,65.65 32.11,65.65 v31.8,65.95 | v21.44,66.11 21.44,76.78 v23.27,78.6 | v26.01,81.35 26.47,81.8 26.47,122.8 39.27,135.6 116.23,135.6 v117.3,134.53
  Bottom 0.305: v31.8,65.95 21.59,65.95 v21.44,66.11 | v23.27,78.6 v26.01,81.35 | v117.3,134.53 117.3,126.1 QUANTUM_CONNECTOR.24
MISO
  Top 0.305: TEENSY3.2_2.12 51.49,79.52 52.68,79.52 53.6,78.6 53.6,74.03 52.81,73.24 50.22,73.24 49.63,72.66 49.63,45.99 50.55,45.08 52.99,45.08 53.75,45.84 53.75,46.45 54.66,47.36 58.02,47.36 58.63,46.75 67.01,46.75 68.38,48.12 68.38,58.49 69.6,59.71 74.78,59.71 75.7,58.79 75.7,57.95 SPI.1
MOSI  (via drill 0.41 pad 0.81)
  Top 0.305: DISPLAY1.SDA 122.65,38.38 116.54,32.27 89.72,32.27 76,45.99 | 76,45.99 57.25,45.99 v56.95,46.3 | v56.95,43.25 56.65,43.55 49.63,43.55 47.81,45.38 47.81,73.4 TEENSY3.2_2.11 | 76,45.99 73.18,48.81 SPI.4
  Bottom 0.305: v56.95,46.3 v56.95,43.25
N$1  (via drill 0.41 pad 0.81)
  Top 0.305: v137.42,24.65 137.42,26.32 LED2.C
  Bottom 0.305: v137.42,24.65 137.42,22.52
  Bottom 0.406: R1.2 137.42,22.52
N$2  (via drill 0.51)
  Top 0.305: LED_5.C 162,64.23 v161.95,64.28
  Bottom 0.305: v161.95,64.28 161.95,61.87 R3.2
N$3  (via drill 0.6)
  Top 0.305: LED5.C 138.89,66.01 v138.79,66.11
  Bottom 0.305: v138.79,66.11 140.64,66.11 R4.2
N$5  (via drill 0.6)
  Top 0.305: v144.58,61.54 144.88,61.23 146.31,61.23 LED6.C
  Bottom 0.305: R11.2 144.76,61.35 v144.58,61.54
N$6  (via drill 0.6)
  Top 0.305: LED7.C v137.87,59.1
  Bottom 0.305: v137.87,59.1 R16.2
N$7  (via drill 0.9 pad 1.68)
  other vias: 178.43,100.49
N$8
  Top 0.813: R5.1 193.83,126.53 LED_RGB.3
N$9  (via drill 0.9 pad 1.68)
  other vias: 203.83,108.11
N$10
  Top 0.813: LED_RGB.1 188.7,128.19 186.95,126.43 R8.1
N$11
  Top 0.813: LED_RGB.2 190.47,124.56 R9.1
N$12  (via drill 0.41 pad 0.81)
  Top 0.305: LED1.C 140.82,26.94 140.82,24.71 v140.77,24.65
  Bottom 0.305: v140.77,24.65 140.77,22.52
  Bottom 0.406: R10.2 140.77,22.52
N$13  (via drill 0.41 pad 0.81)
  Top 0.305: v146.56,24.65 146.56,26.33 LED4.C
  Bottom 0.305: v146.56,24.65 146.56,22.7
  Bottom 0.406: R13.2 146.56,22.7
N$14  (via drill 0.51)
  Top 0.305: v143.36,24.65 LED3.C
  Bottom 0.305: v143.36,24.65 143.36,22.8 R14.2
N$16  (via drill 0.6)
  Top 0.305: v145.49,59.71 LED8.C
  Bottom 0.305: R17.2 v145.49,59.71
N$18
  Bottom 0.406: SW.6 143.84,41.7 R64.2
N$20
  Bottom 0.406: SW.8 137.34,42.15 R62.1
N$21  (via drill 0.9 pad 1.68)
  other vias: 186.05,108.11
N$22  (via drill 0.9 pad 1.68)
  other vias: 186.05,105.57
N$23  (via drill 0.9 pad 1.68)
  other vias: 188.59,105.57
N$24  (via drill 0.9 pad 1.68)
  other vias: 191.13,105.57
N$25  (via drill 0.9 pad 1.68)
  other vias: 193.67,105.57
N$26  (via drill 0.9 pad 1.68)
  other vias: 178.43,95.41
N$27  (via drill 0.9 pad 1.68)
  other vias: 196.21,108.11
N$28  (via drill 0.9 pad 1.68)
  other vias: 196.21,105.57
N$34  (via drill 0.9 pad 1.68)
  other vias: 196.21,103.03
N$35  (via drill 0.9 pad 1.68)
  other vias: 193.67,103.03
N$36  (via drill 0.9 pad 1.68)
  other vias: 191.13,103.03
N$37  (via drill 0.9 pad 1.68)
  other vias: 188.59,103.03
N$38  (via drill 0.9 pad 1.68)
  other vias: 186.05,103.03
N$39  (via drill 0.9 pad 1.68)
  other vias: 186.05,100.49
N$40  (via drill 0.9 pad 1.68)
  other vias: 188.59,100.49
N$41  (via drill 0.9 pad 1.68)
  other vias: 191.13,100.49
N$42  (via drill 0.9 pad 1.68)
  other vias: 193.67,100.49
N$44  (via drill 0.9 pad 1.68)
  other vias: 186.05,92.87
N$45  (via drill 0.9 pad 1.68)
  other vias: 186.05,95.41
N$51  (via drill 0.9 pad 1.68)
  other vias: 191.13,95.41
N$52  (via drill 0.9 pad 1.68)
  other vias: 188.59,95.41
N$54  (via drill 0.9 pad 1.68)
  other vias: 188.59,92.87
N$57  (via drill 0.9 pad 1.68)
  other vias: 191.13,92.87
N$61  (via drill 0.9 pad 1.68)
  other vias: 193.67,92.87
N$62  (via drill 0.9 pad 1.68)
  other vias: 193.67,95.41
N$64  (via drill 0.9 pad 1.68)
  other vias: 196.21,92.87
N$65  (via drill 0.9 pad 1.68)
  other vias: 196.21,95.41
N$66  (via drill 0.9 pad 1.68)
  other vias: 196.21,97.95
N$67  (via drill 0.9 pad 1.68)
  other vias: 196.21,100.49
N$68  (via drill 0.9 pad 1.68)
  other vias: 193.67,97.95
N$81  (via drill 0.9 pad 1.68)
  other vias: 191.13,97.95
N$92  (via drill 0.9 pad 1.68)
  other vias: 188.59,97.95
N$93  (via drill 0.9 pad 1.68)
  other vias: 186.05,97.95
N$94  (via drill 0.9 pad 1.68)
  other vias: 178.43,97.95
N$95  (via drill 0.9 pad 1.68)
  other vias: 191.13,108.11
N$96
  Bottom 0.406: SW.5 147.07,42.38 R6.1
N$97
  Bottom 0.406: SW.7 140.47,41.57 140.47,44.16 140.62,44.31 R63.2
N$98  (via drill 0.9 pad 1.68)
  other vias: 178.43,105.57
N$133  (via drill 0.9 pad 1.68)
  other vias: 178.43,103.03
N$134  (via drill 0.9 pad 1.68)
  other vias: 180.97,108.11
N$135  (via drill 0.9 pad 1.68)
  other vias: 183.51,108.11
N$136  (via drill 0.9 pad 1.68)
  other vias: 180.97,105.57
N$137  (via drill 0.9 pad 1.68)
  other vias: 178.43,108.11
N$138  (via drill 0.9 pad 1.68)
  other vias: 206.37,108.11
N$139  (via drill 0.9 pad 1.68)
  other vias: 183.51,105.57
N$140  (via drill 0.9 pad 1.68)
  other vias: 183.51,103.03
N$141  (via drill 0.9 pad 1.68)
  other vias: 180.97,103.03
N$142  (via drill 0.9 pad 1.68)
  other vias: 201.29,108.11
N$143  (via drill 0.9 pad 1.68)
  other vias: 193.67,108.11
N$144  (via drill 0.9 pad 1.68)
  other vias: 188.59,108.11
N$145  (via drill 0.9 pad 1.68)
  other vias: 203.83,110.65
N$146  (via drill 0.9 pad 1.68)
  other vias: 198.75,110.65
N$147  (via drill 0.9 pad 1.68)
  other vias: 178.43,92.87
N$148  (via drill 0.9 pad 1.68)
  other vias: 180.97,100.49
N$149  (via drill 0.9 pad 1.68)
  other vias: 191.13,110.65
N$150  (via drill 0.9 pad 1.68)
  other vias: 186.05,110.65
N$151  (via drill 0.9 pad 1.68)
  other vias: 196.21,110.65
N$155  (via drill 0.9 pad 1.68)
  other vias: 206.37,110.65
N$157  (via drill 0.9 pad 1.68)
  other vias: 201.29,110.65
N$159  (via drill 0.9 pad 1.68)
  other vias: 180.97,92.87
N$160  (via drill 0.9 pad 1.68)
  other vias: 180.97,95.41
N$162  (via drill 0.9 pad 1.68)
  other vias: 183.51,92.87
N$163  (via drill 0.9 pad 1.68)
  other vias: 183.51,95.41
N$164  (via drill 0.9 pad 1.68)
  other vias: 183.51,97.95
N$165  (via drill 0.9 pad 1.68)
  other vias: 183.51,100.49
N$166  (via drill 0.9 pad 1.68)
  other vias: 180.97,97.95
N$167  (via drill 0.9 pad 1.68)
  other vias: 193.67,110.65
N$168  (via drill 0.9 pad 1.68)
  other vias: 188.59,110.65
N$276  (via drill 0.9 pad 1.68)
  other vias: 198.75,108.11
N$277  (via drill 0.9 pad 1.68)
  other vias: 198.75,105.57
N$278  (via drill 0.9 pad 1.68)
  other vias: 201.29,105.57
N$279  (via drill 0.9 pad 1.68)
  other vias: 203.83,105.57
N$280  (via drill 0.9 pad 1.68)
  other vias: 206.37,105.57
N$285  (via drill 0.9 pad 1.68)
  other vias: 206.37,103.03
N$286  (via drill 0.9 pad 1.68)
  other vias: 203.83,103.03
N$287  (via drill 0.9 pad 1.68)
  other vias: 201.29,103.03
N$288  (via drill 0.9 pad 1.68)
  other vias: 198.75,103.03
N$289  (via drill 0.9 pad 1.68)
  other vias: 198.75,100.49
N$290  (via drill 0.9 pad 1.68)
  other vias: 201.29,100.49
N$291  (via drill 0.9 pad 1.68)
  other vias: 203.83,100.49
N$292  (via drill 0.9 pad 1.68)
  other vias: 206.37,100.49
N$294  (via drill 0.9 pad 1.68)
  other vias: 198.75,92.87
N$295  (via drill 0.9 pad 1.68)
  other vias: 198.75,95.41
N$296  (via drill 0.9 pad 1.68)
  other vias: 203.83,95.41
N$297  (via drill 0.9 pad 1.68)
  other vias: 201.29,95.41
N$299  (via drill 0.9 pad 1.68)
  other vias: 201.29,92.87
N$301  (via drill 0.9 pad 1.68)
  other vias: 203.83,92.87
N$303  (via drill 0.9 pad 1.68)
  other vias: 206.37,92.87
N$304  (via drill 0.9 pad 1.68)
  other vias: 206.37,95.41
N$310  (via drill 0.9 pad 1.68)
  other vias: 206.37,97.95
N$311  (via drill 0.9 pad 1.68)
  other vias: 203.83,97.95
N$312  (via drill 0.9 pad 1.68)
  other vias: 201.29,97.95
N$313  (via drill 0.9 pad 1.68)
  other vias: 198.75,97.95
PALLA  (via drill 0.41)
  Top 0.305: TEENSY3.2_2.28 43.34,77.03 42.01,75.71 34.09,75.71 v33.94,75.86 | v32.87,84.24 32.57,84.55 32.57,118.84 42.17,128.44 102.34,128.44 103.36,127.42 103.36,124.81 QUANTUM_CONNECTOR.13
  Bottom 0.305: v33.94,75.86 33.94,78.15 34.24,78.45 34.24,82.87 v32.87,84.24
PROGRAM
  Top 0.406: PROGRAM.A2 64.42,24.22 64.42,37.15 62.79,38.78 USB_2.5
PULS  (via drill 0.41)
  Top 0.305: TEENSY3.2_2.23/A9 36.2,53.64 37.9,51.93 43.39,51.93 44.3,51.02 44.3,43.09 v43.84,42.64 | v45.06,39.28 45.98,38.37 54.66,38.37 57.1,35.93 57.1,23.44 59.69,20.84 158.3,20.84 161.34,23.89 161.34,33.34 166.83,38.83 166.83,41.27 165.76,42.33 159.21,42.33 158.14,41.27 158.14,40.12 ENCODER.B
  Bottom 0.305: v43.84,42.64 43.84,40.5 v45.06,39.28
  Bottom 0.813: ENCODER.B 156.36,41.77 C57.2
PWM1
  Top 0.305: TEENSY3.2_2.5 51.49,61.84 55.73,61.84 69.6,75.71 69.6,98.72 90.66,119.78 90.66,124.91 91.82,126.08 QUANTUM_CONNECTOR.4
PWM2  (via drill 0.41 pad 0.81)
  Top 0.305: TEENSY3.2_2.9 51.69,72.2 55.58,72.2 57.71,74.34 v57.71,81.96 | v67.47,91.25 68.08,91.86 68.08,99.33 80.11,111.37 80.11,111.67 81.49,113.05 v82.55,113.05 | v91.54,115.48 97.18,115.48 98.25,116.55 98.25,124.78 QUANTUM_CONNECTOR.10
  Bottom 0.305: v82.55,113.05 90.48,113.05 91.54,114.11 v91.54,115.48 | v57.71,81.96 67.01,91.25 v67.47,91.25
PWM3  (via drill 0.41)
  Top 0.305: TEENSY3.2_2.32 38.26,69.41 36.99,70.68 v31.96,70.68 | v101.3,136.67 100.99,136.36 38.97,136.36 25.71,123.1 25.71,83.63 20.53,78.45 20.53,72.2 v19.92,71.59
  Bottom 0.305: v101.3,136.67 101.3,127.83 100.84,127.37 100.84,124.83 QUANTUM_CONNECTOR.9 | v31.96,70.68 20.83,70.68 v19.92,71.59
PWM4
  Top 0.305: TEENSY3.2_2.4 55.73,59.25 70.36,73.88 70.36,98.42 91.93,119.98 QUANTUM_CONNECTOR.3
RED  (via drill 0.41 pad 0.81, 0.9 pad 1.68)
  Top 0.305: TEENSY3.2_2.20/A6 31.85,61.79 27.23,66.41 27.23,122.19 39.42,134.38 57.71,134.38 58.32,134.99 60.76,134.99 62.28,133.47 118.21,133.47 121.11,136.36 130.1,136.36 133.45,133.01 133.45,115.79 135.89,113.35 175.36,113.35 v176.58,114.57 | v180.85,117.31 180.85,115.94 181,115.79
  Top 0.813: R9.2 190.44,120.04 188.32,117.92 182.98,117.92 181,115.94 181,115.79 181,110.66 v181.02,110.65
  Bottom 0.305: v176.58,114.57 179.48,114.57 179.94,115.03 179.94,116.4 v180.85,117.31
SCK  (via drill 0.41, 0.41 pad 0.81)
  Top 0.305: DISPLAY1.SCK 129.38,40.92 131.17,39.13 131.17,30.9 129.8,29.53 124.16,29.53 123.7,29.99 88.65,29.99 74.93,43.7 | 74.93,43.7 58.47,43.7 58.02,43.25 58.02,42.64 57.71,41.42 33.94,41.42 30.28,45.08 30.28,53.46 25.4,58.33 v25.4,76.32 | v33.23,79.57 TEENSY3.2_2.13 | 74.93,43.7 74.17,42.94 v74.17,42.64 | v72.95,47.06 71.89,48.12 71.91,53.13 71.91,56.91 72.93,57.93 SPI.3
  Bottom 0.305: v74.17,42.64 72.95,43.86 v72.95,47.06 | v33.23,79.57 28.65,79.57 v25.4,76.32
SCL  (via drill 0.41)
  Top 0.305: TEENSY3.2_2.19/A5 30.84,64.33 v30.43,64.74 | v23.57,64.58 23.57,57.73 28.6,52.7 28.6,44.31 33.02,39.89 41.56,39.89 44.76,36.69 53.75,36.69 55.58,34.87 55.58,22.83 61.37,17.03 107.85,17.03 v110.9,19.47 | v111.2,33.19 112.12,34.1 U$5.SCL
  Bottom 0.305: R65.1 108.77,63.21 110.14,63.21 111.03,62.32 111.03,55.52 U$5.SCL | v30.43,64.74 23.73,64.74 v23.57,64.58 | v110.9,19.47 110.9,32.88 v111.2,33.19
SDA  (via drill 0.41)
  Top 0.305: TEENSY3.2_2.18/A4 v28.91,66.87 | v23.27,66.87 22.36,65.95 22.36,57.73 27.69,52.39 27.69,44.01 32.57,39.13 41.1,39.13 44.3,35.93 53.14,35.93 54.66,34.41 54.66,22.67 61.52,15.82 v61.52,15.36 | v70.97,15.36 109.07,15.36 v113.34,19.63 | v110.14,34.87 110.14,52.54 109.68,53 109.68,54.32 U$5.SDA
  Bottom 0.305: 108.49,59.83 R66.1 108.64,55.36 U$5.SDA | v28.91,66.87 v23.27,66.87 | v61.52,15.36 61.52,15.66 62.59,17.03 69.6,17.03 v70.97,15.36 | v113.34,19.63 113.34,33.8 112.58,34.56 110.44,34.56 v110.14,34.87
SEL  (via drill 0.41)
  Top 0.305: TEENSY3.2_2.A11 38.74,58.72 37.44,57.42 37.44,55.9 37.9,55.44 45.22,55.44 46.13,54.52 46.13,43.55 v47.2,42.49 | v49.18,40.5 55.12,40.5 58.63,37 58.63,24.35 60.61,22.37 154.9,22.37 ENCODER.E
  Bottom 0.305: v47.2,42.49 v49.18,40.5
SOLENOIDE
  Top 0.305: TEENSY3.2_2.29 40.01,78.3 32.41,78.3 31.8,78.91 31.8,119.29 41.86,129.35 103.28,129.35 104.65,127.98 104.65,126.1 QUANTUM_CONNECTOR.14
SPEED  (via drill 0.41)
  Top 0.305: TEENSY3.2_2.A12 42.5,60.47 31.8,60.47 26.47,65.8 26.47,77.23 24.18,79.52 v24.18,80.74
  Bottom 0.305: v24.18,80.74 20.37,84.4 19,84.4 18.34,85.06 R12.S
TEENSY1-RX_TEENSY2-TX
  Top 0.305: QUANTUM_CONNECTOR.29 124.95,113.99 124.01,113.05 88.19,113.05 72.65,97.5 72.65,68.55 55.88,51.78 51.59,51.78 TEENSY3.2_2.1
TEENSY1-TX_TEENSY2-RX
  Top 0.305: QUANTUM_CONNECTOR.30 129.57,126.08 131.02,124.63 131.02,116.4 127.05,112.44 88.65,112.44 73.41,97.2 73.41,66.41 56.04,49.04 51.49,49.04 TEENSY3.2_2.0
TONE  (via drill 0.41)
  Top 0.305: TEENSY3.2_2.RESET/DAC 38.74,81.42 38.05,82.11 33.79,82.11 v33.18,81.5 | v24.18,77.38 24.18,73.42 24.64,72.97 24.64,57.88 29.52,53 29.52,44.62 33.48,40.66 41.86,40.66 45.06,37.46 54.21,37.46 56.34,35.32 56.34,23.13 61.67,17.8 105.72,17.8 v107.24,18.86
  Bottom 0.305: v33.18,81.5 28.3,81.5 v24.18,77.38 | v107.24,18.86 107.24,27.35 BUZZER.+
VUSB
  Top 0.305: USB.VBUS 69.35,34.15 72.95,37.76 USB_2.1

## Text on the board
tPlace: The best way to predict the future is to invent it. | Developed by: / / Alessio Di Brigida / Emanuele Giacomini / Andrea Valeri / Fabio Ricci | PWM 25 G | PWM 20 R | PWM 6 B | 5V | GND | 3.3V | GND | 5V | 3.3V | $$$ | 5V | ° | ON | 3.3V
tNames: 1 | 3 | 5 | 7 | 9 | 11 | 13 | 15 | 17 | 19 | 21 | 23 | 25 | 27 | 29 | Inferiore | Program
Reference: posizione esatta

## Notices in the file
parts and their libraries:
SparkFun-DigitalIC: Licensing: Creative Commons ShareAlike 4.0 International - https://creativecommons.org/licenses/by-sa/4.0
